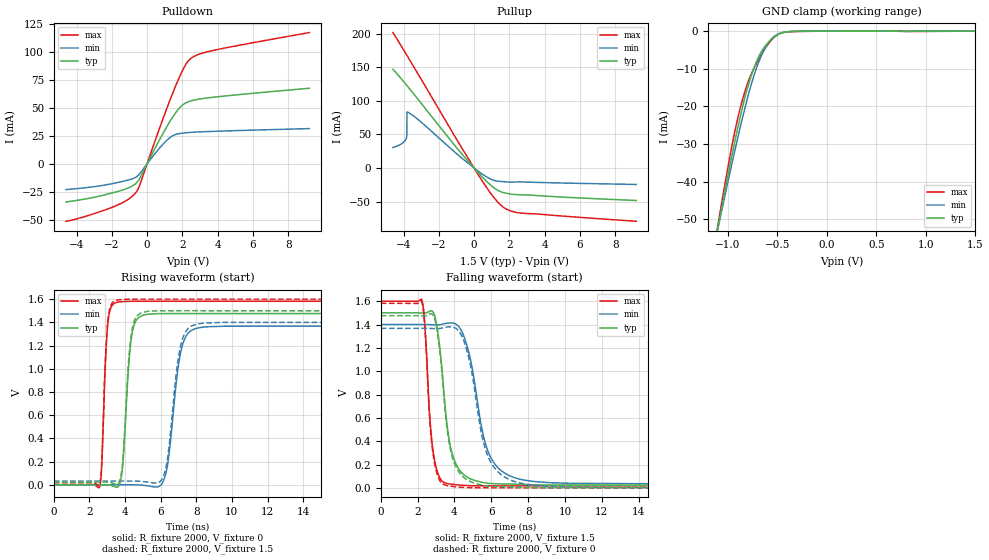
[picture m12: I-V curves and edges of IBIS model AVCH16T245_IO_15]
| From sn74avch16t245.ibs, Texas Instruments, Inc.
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[Model]   AVCH16T245_IO_15
Model_type  I/O
Vinl=0.49
Vinh=1.04
Enable   Active-Low
Vref =   0
Rref =   2000
Cref =   15p
Vmeas =   0.75
| variable   typ   min   max
C_comp   5.30pF   4.64pF   5.87pF
| C_pullup   5.22pF   3.72pF   7.64pF
| C_pulldown   4.91pF   4.33pF   5.57pF
| C_tri-state   5.30pF   4.64pF   5.87pF
[Temperature Range]   40   100   -40
| Ambient temperature   25   85   -40
[Voltage range]   1.5   1.4   1.6
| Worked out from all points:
|   slope of the pulldown table from 0 to 0.225 V, typ, clamps not added: 32.1 ohm
|   slope of the pullup table from 0 to 0.225 V, typ, clamps not added: 33.9 ohm
|   GND clamp passes 1 mA (typ) near -0.50 V on its own axis
|   rising waveform, R_fixture 2000, V_fixture 0: 20-80 % time 361ps typ, 590ps min, 241ps max; typ from 0 V to 1.48 V
|   falling waveform, R_fixture 2000, V_fixture 1.5: 20-80 % time 635ps typ, 1.01ns min, 388ps max; typ from 1.5 V to 0.023 V
|   rising waveform, R_fixture 2000, V_fixture 1.5: 20-80 % time 357ps typ, 576ps min, 239ps max; typ from 0.023 V to 1.5 V
|   falling waveform, R_fixture 2000, V_fixture 0: 20-80 % time 635ps typ, 1.01ns min, 381ps max; typ from 1.48 V to 0 V
[GND Clamp]
| AVCH16T245_IO_15
|   Voltage   I(typ)   I(min)   I(max)
-4.6V     -599.6mA   -548.2mA   -664.6mA
-1.1V     -52.36mA   -52.8mA    -51.85mA
-1.075V   -48.9mA    -49.67mA   -47.95mA
-930mV    -29.68mA   -32.07mA   -27.01mA
-880mV    -23.6mA    -26.34mA   -21.2mA
-830mV    -18.08mA   -20.9mA    -16.41mA
-765mV    -12.13mA   -14.48mA   -11.64mA
-685mV    -6.738mA   -8.147mA   -7.41mA
-605mV    -3.434mA   -3.729mA   -3.946mA
-535mV    -1.679mA   -1.475mA   -1.741mA
-370mV    -121.9uA   -99.54uA   -128.4uA
1.5V      812.2pA    1.554uA    -44.11nA
[Pulldown]
| AVCH16T245_IO_15
|   Voltage   I(typ)   I(min)   I(max)
-4.6V     -34.07mA   -23.01mA   -51.35mA
-1.88V    -25.6mA    -17.43mA   -38.2mA
-1.09V    -21.68mA   -14.59mA   -31.97mA
-625mV    -17.31mA   -11.83mA   -25.44mA
-415mV    -12.94mA   -8.777mA   -18.95mA
595mV     18.22mA    11.97mA    26.91mA
1.265V    37.01mA    23.01mA    55.56mA
1.695V    47.18mA    26.54mA    72.43mA
2.025V    52.71mA    27.44mA    83.88mA
2.495V    56.22mA    28.09mA    94.25mA
3.835V    59.62mA    29.04mA    101.6mA
9.2V      67.51mA    31.46mA    117.2mA
[Pullup]
| AVCH16T245_IO_15
|   Voltage   I(typ)   I(min)   I(max)
-4.6V     146.8mA    30.47mA    201.5mA
-4.1V     131.8mA    36.24mA    180.2mA
-3.85V    123.9mA    43.96mA    169.4mA
-3.81V    122.6mA    49.37mA    167.6mA
-3.805V   122.5mA    83.3mA     167.4mA
-3.785V   121.8mA    83.17mA    166.5mA
-3.155V   101.3mA    71.56mA    138.9mA
175mV     -5.197mA   -3.574mA   -7.497mA
980mV     -26.35mA   -16.94mA   -39.04mA
1.625V    -36.35mA   -20.39mA   -57.65mA
2.595V    -39.89mA   -20.78mA   -66.9mA
9.2V      -48.41mA   -24.54mA   -79.36mA
[Ramp]
| AVCH16T245_IO_15
| variable   typ   min   max
dV/dt_r   0.90/3.76E-10   0.83/5.98E-10   0.96/2.56E-10
dV/dt_f   0.90/6.42E-10   0.83/1.02E-09   0.96/3.95E-10
R_load = 2000
[Rising Waveform]
| AVCH16T245_IO_15
R_fixture =   2000
C_fixture =   0
L_fixture =   0
V_fixture =   0
V_fixture_min = 0
V_fixture_max = 0
|   Time   V(typ)   V(min)   V(max)
0s        19.41nV    97.7nV     527.2pV
2.575ns   904.3uV    -139.8uV   -16.3mV
3.01ns    -56.85uV   130.7uV    1.349V
3.475ns   -18.78mV   607.2uV    1.569V
4.38ns    1.289V     545.3uV    1.581V
4.98ns    1.46V      -3.079mV   1.582V
6.22ns    1.475V     60.26mV    1.582V
7.11ns    1.476V     1.131V     1.582V
7.91ns    1.476V     1.344V     1.582V
29.99ns   1.476V     1.367V     1.582V
[Falling Waveform]
| AVCH16T245_IO_15
R_fixture =   2000
C_fixture =   0
L_fixture =   0
V_fixture =   1.5
V_fixture_min = 1.4
V_fixture_max = 1.6
|   Time   V(typ)   V(min)   V(max)
0s        1.5V       1.4V       1.6V
2.225ns   1.499V     1.4V       1.612V
2.81ns    1.512V     1.398V     348.5mV
3.14ns    1.284V     1.398V     107.1mV
3.51ns    667.7mV    1.409V     41.09mV
3.855ns   306.1mV    1.413V     31.11mV
4.39ns    129.6mV    1.343V     22.59mV
5.785ns   40.44mV    327.3mV    17.32mV
7.265ns   31.05mV    86.78mV    17.13mV
29.99ns   23.4mV     32.34mV    17.1mV
[Rising Waveform]
| AVCH16T245_IO_15
R_fixture =   2000
C_fixture =   0
L_fixture =   0
V_fixture =   1.5
V_fixture_min = 1.4
V_fixture_max = 1.6
|   Time   V(typ)   V(min)   V(max)
0s        23.4mV     32.34mV    17.1mV
2.575ns   24.29mV    32.21mV    1.45mV
3.005ns   23.31mV    32.49mV    1.365V
3.485ns   4.624mV    32.95mV    1.589V
4.365ns   1.31V      32.72mV    1.599V
4.96ns    1.485V     29.33mV    1.6V
6.2ns     1.5V       92.47mV    1.6V
7.08ns    1.5V       1.17V      1.6V
7.87ns    1.5V       1.377V     1.6V
29.99ns   1.5V       1.4V       1.6V
[Falling Waveform]
| AVCH16T245_IO_15
R_fixture =   2000
C_fixture =   0
L_fixture =   0
V_fixture =   0
V_fixture_min = 0
V_fixture_max = 0
|   Time   V(typ)   V(min)   V(max)
0s        1.476V     1.367V     1.582V
2.225ns   1.474V     1.367V     1.593V
2.805ns   1.487V     1.365V     328.4mV
3.125ns   1.273V     1.365V     88.12mV
3.495ns   656.9mV    1.376V     23.49mV
3.82ns    301.9mV    1.379V     13.76mV
4.38ns    108.1mV    1.307V     4.92mV
5.74ns    16.98mV    302.9mV    206uV
7.245ns   7.238mV    54.9mV     22.57uV
29.99ns   470.8nV    3.572uV    218.8nV
